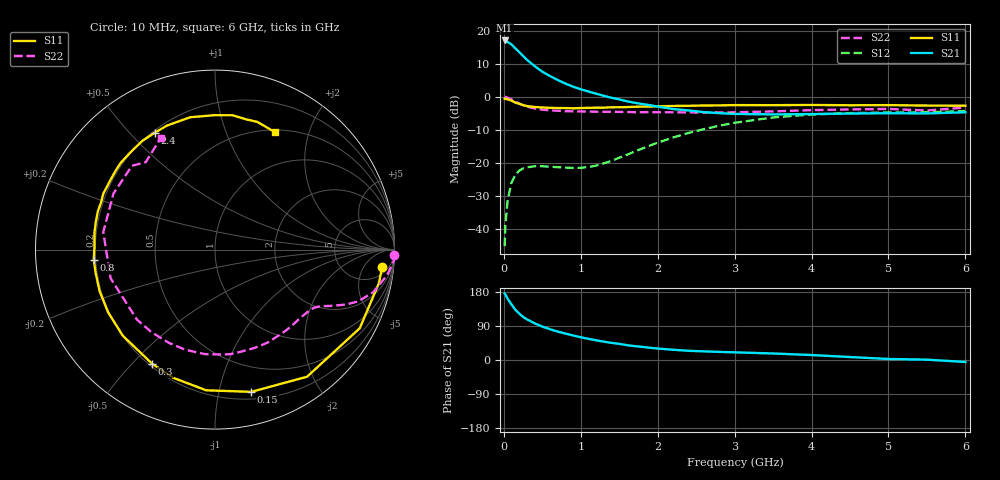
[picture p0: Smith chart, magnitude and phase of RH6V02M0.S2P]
! SIEMENS Small Signal Semiconductors
! BFR106
! Si NPN RF Bipolar Junction Transistor in SOT23
! VCE = 6 V  IC = 2 mA
! Common Emitter S-Parameters:  August  1996
# GHz  S  MA  R  50
!  f  S11  S21  S12  S22
! GHz  MAG  ANG  MAG  ANG  MAG  ANG  MAG  ANG
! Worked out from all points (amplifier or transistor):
!   36 points, 10 MHz to 6 GHz, reference 50 ohm
!   highest |S21| = 17.0 dB at 10 MHz (marker M1)
!   |S21| within 3 dB of that: start of sweep to 177.4 MHz
!   unconditionally stable (mu >= 1): 782.4 MHz to 1.832 GHz; 4.08 GHz to end of sweep
!   at 250 MHz: K = 0.32, MSG = 17.0 dB, |S12| = -21.6 dB
!   at 1.4 GHz: K = 1.24, MAG = 6.6 dB, |S12| = -19.3 dB
!   at 6 GHz: K = 1.02, MAG = -1.1 dB, |S12| = -4.3 dB
!   S11 on the Smith chart (normalised r, x): 10 MHz: 9, -14; 150 MHz: 0.26, -1.25; 300 MHz: 0.21, -0.57; 800 MHz: 0.19, -0.04; 2.4 GHz: 0.21, +0.59; 6 GHz: 0.53, +1.50
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0.01  0.9361 -6.0  7.083 175.6  0.0056 88.3  0.9991 -1.7
0.02  0.9321 -11.6  7.02 172.8  0.0114 82.9  0.9984 -3.6
0.05  0.9179 -28.5  6.725 161.4  0.028 74.8  0.9701 -8.4
0.1  0.8745 -54.1  6.159 146.4  0.051 61.7  0.9125 -15.1
0.15  0.8179 -75.7  5.378 132.3  0.0668 50.7  0.8481 -19.9
0.2  0.7854 -93.6  4.734 122.6  0.0772 43.9  0.7924 -22.7
0.25  0.7513 -107.9  4.134 113.6  0.0832 37.7  0.7443 -24.7
0.3  0.7262 -118.8  3.619 107.3  0.0864 34.2  0.7112 -26.2
0.4  0.7029 -136.9  2.906 96.9  0.0898 29.2  0.6672 -28.2
0.5  0.6907 -149.7  2.397 88.2  0.0899 27.3  0.6409 -30.3
0.6  0.6833 -160.2  2.059 81.2  0.0882 27.5  0.6257 -32.9
0.8  0.6779 -175.2  1.586 69.8  0.0858 31.8  0.6084 -38.6
1.1  0.6817 166.9  1.201 55.9  0.0876 47.1  0.5993 -48.7
1.6  0.7013 145.1  0.856 39.2  0.1338 69.6  0.5904 -68.2
2.2  0.7285 123.9  0.655 27.0  0.2437 70.9  0.5849 -95.6
2.4  0.7326 117.3  0.624 24.3  0.2852 67.7  0.582 -106.4
3  0.7502 100.6  0.553 20.2  0.406 54.9  0.5841 -138.1
3.5  0.7487 90.5  0.543 17.2  0.4886 42.6  0.6031 -164.6
4.5  0.7462 76.7  0.56 7.8  0.5684 19.8  0.6462 151.1
5  0.7496 71.6  0.566 2.7  0.5812 11.1  0.6571 134.7
5.5  0.7386 66.5  0.562 0.9  0.5835 6.8  0.6215 128.4
6  0.7347 62.9  0.585 -5.2  0.6105 -1.4  0.6904 116.0
